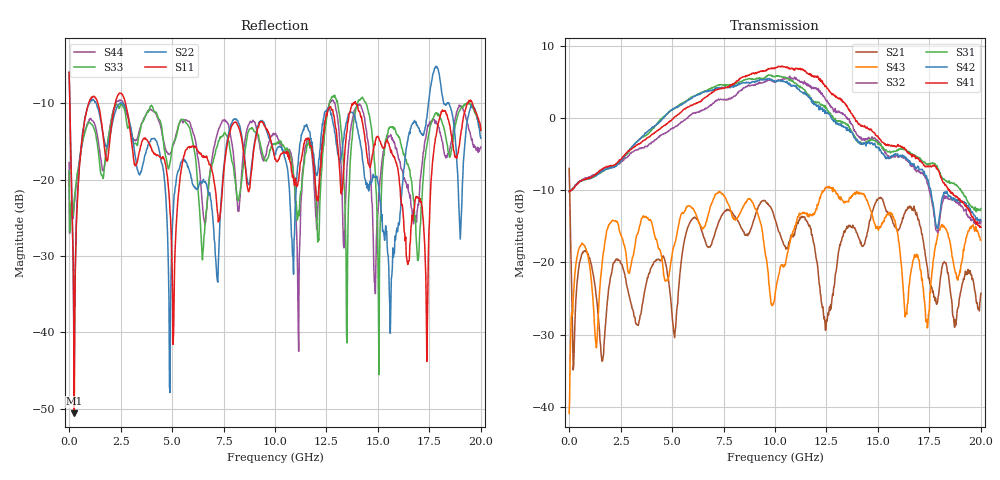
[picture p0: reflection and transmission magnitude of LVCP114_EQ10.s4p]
!Agilent Technologies,N5230A,MY46400459,A.07.50.48
!Agilent N5230A: A.07.50.48
!Date: Monday, January 09, 2012 14:02:34
!Correction: S11(Full 4 Port(1,2,3,4))
!S12(Full 4 Port(1,2,3,4))
!S13(Full 4 Port(1,2,3,4))
!S14(Full 4 Port(1,2,3,4))
!S21(Full 4 Port(1,2,3,4))
!S22(Full 4 Port(1,2,3,4))
!S23(Full 4 Port(1,2,3,4))
!S24(Full 4 Port(1,2,3,4))
!S31(Full 4 Port(1,2,3,4))
!S32(Full 4 Port(1,2,3,4))
!S33(Full 4 Port(1,2,3,4))
!S34(Full 4 Port(1,2,3,4))
!S41(Full 4 Port(1,2,3,4))
!S42(Full 4 Port(1,2,3,4))
!S43(Full 4 Port(1,2,3,4))
!S44(Full 4 Port(1,2,3,4))
!S4P File: Measurements: <S11,S12,S13,S14>,
!<S21,S22,S23,S24>,
!<S31,S32,S33,S34>,
!<S41,S42,S43,S44>:
# Hz S  dB  R 50
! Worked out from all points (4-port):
!   801 points, 300 kHz to 20 GHz, reference 50 ohm
!   strongest paths, dB at 300 kHz, 5 GHz, 10 GHz, 15 GHz, 20 GHz:
!     S41: -10.2, -0.2, 6.9, -2.5, -15.1
!     S42: -10.2, 1.1, 5.1, -4.1, -14.2
!     S31: -10.2, 1.2, 5.7, -3.6, -12.5
!     S32: -10.1, -1.5, 4.9, -3.4, -14.3
!     S43: -40.9, -19.0, -24.5, -15.2, -16.9
!     S21: -7.0, -27.2, -14.0, -11.2, -24.3
!   lowest |S11| = -50.6 dB at 250.3 MHz (marker M1), VSWR 1.01, Z = 50.3 - j0.0174 ohm
!   |S11| at or under -10 dB: 34.46 MHz to 952.7 MHz (918.2 MHz wide, 186 % of centre); 2.737 GHz to 13.8 GHz (11.06 GHz wide, 134 % of centre); 13.92 GHz to 19.34 GHz (5.425 GHz wide, 32.6 % of centre)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
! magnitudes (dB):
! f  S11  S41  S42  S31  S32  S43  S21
! 300 kHz  -6.0  -10.2  -10.2  -10.2  -10.1  -40.9  -7.0
! 250.3 MHz  -50.6  -9.6  -9.6  -9.7  -9.6  -22.7  -31.3
! 1.15 GHz  -9.1  -8.1  -8.1  -8.2  -7.9  -24.8  -21.4
! 4.9 GHz  -24.1  -0.4  0.9  1.0  -1.7  -20.9  -24.2
! 8.025 GHz  -12.5  4.8  4.5  4.6  3.0  -14.0  -13.7
! 17.35 GHz  -37.4  -6.7  -8.0  -6.4  -8.4  -28.2  -19.9
! 20 GHz  -13.5  -15.1  -14.2  -12.5  -14.3  -16.9  -24.3
